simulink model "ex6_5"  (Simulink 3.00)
settings: Solver=VariableStepDiscrete  SolverMode=SingleTasking  StartTime=0.0  StopTime=20  RelTol=1e-3  AbsTol=1e-6

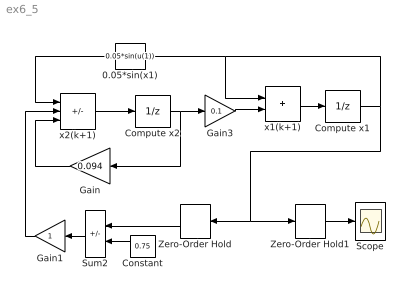
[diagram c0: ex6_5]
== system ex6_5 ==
  0.05*sin(x1) : Fcn  Orientation=left  Expr=0.05*sin(u(1))
  Compute x1 : UnitDelay  X0=0  SampleTime=0.1
  Compute x2 : UnitDelay  X0=0  SampleTime=0.1
  Constant : Constant  Orientation=left  Value=0.75
  Gain : Gain  Orientation=left  Gain=0.094  SaturateOnIntegerOverflow=on
  Gain1 : Gain  Orientation=left  Gain=1  SaturateOnIntegerOverflow=on
  Gain3 : Gain  Gain=0.1  SaturateOnIntegerOverflow=on
  Scope : Scope
  Sum2 : Sum  Orientation=left  Inputs=-+  SaturateOnIntegerOverflow=on
  Zero-Order Hold : ZeroOrderHold  Orientation=left  SampleTime=0.25
  Zero-Order Hold1 : ZeroOrderHold  SampleTime=0.5
  x1(k+1) : Sum  Inputs=++  SaturateOnIntegerOverflow=on
  x2(k+1) : Sum  Inputs=-++  SaturateOnIntegerOverflow=on
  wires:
  x2(k+1)/1 -> Compute x2/1
  Gain/1 -> x2(k+1)/3
  0.05*sin(x1)/1 -> x2(k+1)/1
  Gain3/1 -> x1(k+1)/2
  x1(k+1)/1 -> Compute x1/1
  Compute x1/1 -> 0.05*sin(x1)/1, x1(k+1)/1, Zero-Order Hold1/1, Zero-Order Hold/1
  Zero-Order Hold1/1 -> Scope/1
  Gain1/1 -> x2(k+1)/2
  Sum2/1 -> Gain1/1
  Zero-Order Hold/1 -> Sum2/1
  Constant/1 -> Sum2/2
  Compute x2/1 -> Gain3/1, Gain/1
